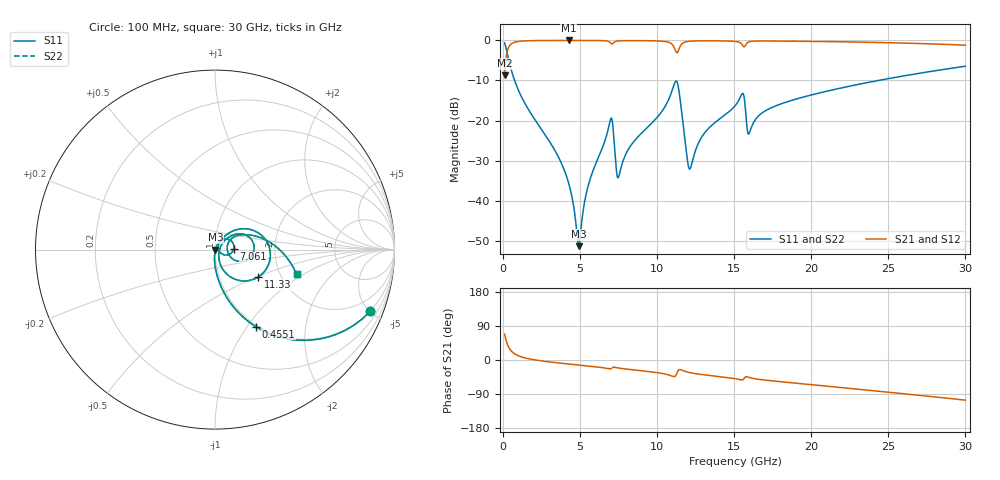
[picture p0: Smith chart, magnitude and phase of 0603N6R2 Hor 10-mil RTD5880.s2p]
# GHz S MA R 50
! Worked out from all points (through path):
!   3201 points, 100 MHz to 30 GHz, reference 50 ohm
!   highest |S21| = -0.02 dB at 4.267 GHz (marker M1); lowest = -8.7 dB at 100 MHz (marker M2)
!   group delay of S21, straight-line fit = 10.5 ps
!   lowest |S11| = -51.3 dB at 4.912 GHz (marker M3), VSWR 1.01, Z = 50.3 - j0.0634 ohm
!   |S11| at or under -10 dB: 746.8 MHz to 24.35 GHz (23.61 GHz wide, 188 % of centre)
!   |S22| runs from -51.3 to -0.6 dB; largest |S21 - S12| = 0
!   S11 on the Smith chart (normalised r, x): 100 MHz: 0.98, -5.03; 455.1 MHz: 0.98, -1.10; 7.061 GHz: 1.23, +0.00; 11.33 GHz: 1.53, -0.51; 30 GHz: 2.45, -0.87
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0.1  0.9306 -21.7  0.3659 68.3  0.3659 68.3  0.9306 -21.7
0.4550625  0.4849 -62.2  0.8739 27.8  0.8739 27.8  0.4849 -62.2
1.258625  0.1867 -82.3  0.9812 7.3  0.9812 7.3  0.1867 -82.3
4.267313  0.01629 -92.2  0.9974 -10.7  0.9974 -10.7  0.01629 -92.2
4.912031  0.002716 -13.4  0.9972 -13.4  0.9972 -13.4  0.002716 -13.4
5.089563  0.00516 42.7  0.9971 -14.1  0.9971 -14.1  0.00516 42.7
5.6315  0.01817 63.1  0.9964 -16.4  0.9964 -16.4  0.01817 63.1
7.061094  0.1042 0.9  0.9028 -21.5  0.9028 -21.5  0.1042 0.9
7.50025  0.01992 23.9  0.9857 -21.2  0.9857 -21.2  0.01992 23.9
8.266438  0.0481 57.8  0.9929 -25.2  0.9929 -25.2  0.0481 57.8
10.06978  0.1137 50.9  0.9829 -33.8  0.9829 -33.8  0.1137 50.9
10.94809  0.2307 28.7  0.9003 -42.2  0.9003 -42.2  0.2307 28.7
11.33119  0.2855 -32.2  0.7145 -30.0  0.7145 -30.0  0.2855 -32.2
12.11606  0.02488 -10.1  0.9769 -33.3  0.9769 -33.3  0.02488 -10.1
13.05044  0.06903 42.8  0.9878 -39.1  0.9878 -39.1  0.06903 42.8
15.05  0.1527 34.8  0.9721 -49.2  0.9721 -49.2  0.1527 34.8
15.55456  0.2184 3.8  0.861 -52.2  0.861 -52.2  0.2184 3.8
15.98438  0.07031 14.0  0.9631 -46.3  0.9631 -46.3  0.07031 14.0
17.04022  0.133 33.4  0.9829 -53.2  0.9829 -53.2  0.133 33.4
20.03956  0.2095 23.0  0.9712 -65.3  0.9712 -65.3  0.2095 23.0
25.01978  0.3339 3.7  0.9352 -85.0  0.9352 -85.0  0.3339 3.7
30  0.4758 -16.9  0.8711 -105.9  0.8711 -105.9  0.4758 -16.9
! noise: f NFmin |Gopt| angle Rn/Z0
0.1  0.0003653  0.9347  0.6086  0.001246
3.417  0.003959  0.8066  9.391  0.004229
6.743  0.01592  0.9006  18.35  0.03414
10.06  0.01511  0.8489  27.18  0.02012
13.39  0.01585  0.8136  35.97  0.01608
16.7  0.01846  0.8034  44.52  0.01674
20.03  0.01667  0.7497  52.65  0.01083
23.35  0.0187  0.7439  60.66  0.011
26.67  0.02114  0.7444  68.5  0.01146
30  0.02387  0.7482  76.14  0.01197
